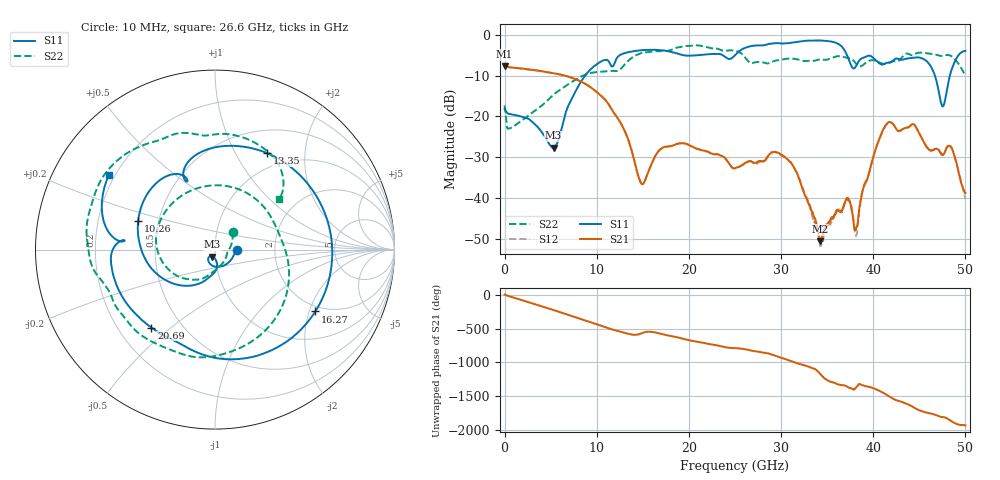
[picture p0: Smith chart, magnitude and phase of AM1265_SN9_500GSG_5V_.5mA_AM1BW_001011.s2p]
!Keysight Technologies,N5245B,MY58422270,A.16.20.02
!Date: Thursday, March 05, 2026 00:38:12
!Correction: S11(C  2-Port  )
!S21(C  2-Port  )
!S12(C  2-Port  )
!S22(C  2-Port  )
!S2P File: Measurements: S11, S21, S12, S22:
# Hz S  dB  R 50
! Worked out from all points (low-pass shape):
!   3201 points, 10 MHz to 50 GHz, reference 50 ohm
!   highest |S21| = -7.68 dB at 10 MHz (marker M1); lowest = -50.6 dB at 34.22 GHz (marker M2)
!   |S21| within 3 dB of the highest: start of sweep to 7.513 GHz
!   lowest |S11| = -27.7 dB at 5.321 GHz (marker M3), VSWR 1.09, Z = 48.4 - j3.74 ohm
!   |S11| at or under -10 dB: start of sweep to 8.743 GHz; 46.69 GHz to 48.31 GHz (1.617 GHz wide, 3.4 % of centre)
!   |S22| runs from -23.0 to -2.6 dB; largest |S21 - S12| = 0.007
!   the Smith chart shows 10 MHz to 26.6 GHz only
!   S11 on the Smith chart (normalised r, x): 10 MHz: 1.28, -0.00; 10.26 GHz: 0.38, +0.15; 13.35 GHz: 0.79, +1.36; 16.27 GHz: 1.82, -2.20; 20.69 GHz: 0.34, -0.43; 26.6 GHz: 0.18, +0.31
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1e7  -18.16 -0.4  -7.68 3.3  -7.65 2.4  -17.28 44.5
2.290794e9  -20.32 -84.1  -8.35 -96.8  -8.36 -96.8  -20.32 -74.6
5.321438e9  -27.67 -111.0  -9.41 134.1  -9.41 134.2  -14.65 -116.9
8.352081e9  -11.27 -132.9  -11.51 -2.7  -11.50 -2.6  -10.16 -172.5
1.025795e10  -6.81 159.8  -14.48 -89.1  -14.47 -89.2  -9.05 125.2
1.335108e10  -4.28 61.5  -25.22 145.3  -25.26 145.3  -6.52 -33.2
1.488202e10  -3.76 10.8  -36.54 150.3  -36.46 150.3  -4.38 -96.3
1.627237e10  -3.65 -31.6  -30.06 165.6  -30.01 166.1  -3.99 -133.6
1.667854e10  -3.69 -43.4  -28.58 153.0  -28.54 153.4  -4.02 -142.3
2.069336e10  -5.03 -129.2  -27.75 30.3  -27.75 30.6  -2.57 148.4
2.5005e10  -4.97 173.6  -32.72 -68.3  -32.65 -69.0  -3.90 71.2
2.659843e10  -2.83 145.1  -30.94 -99.8  -30.98 -99.4  -6.80 38.4
3.066012e10  -2.06 78.5  -30.42 120.2  -30.41 120.6  -5.85 -54.7
3.334708e10  -1.39 35.6  -43.33 -2.0  -44.17 -2.9  -6.35 -127.9
3.422191e10  -1.38 20.5  -50.56 -85.5  -51.05 -79.2  -6.01 -146.3
3.717444e10  -5.08 -41.1  -40.04 82.4  -40.52 82.0  -5.63 156.4
3.815862e10  -7.57 -22.8  -47.26 71.3  -49.12 63.0  -7.14 139.3
4.167354e10  -6.82 -54.6  -21.38 -57.5  -21.35 -57.7  -6.82 114.2
4.511035e10  -5.61 -102.6  -24.60 86.8  -24.65 86.5  -4.35 75.0
4.654757e10  -9.09 -152.5  -28.13 35.0  -28.24 34.5  -4.73 53.8
4.770358e10  -16.86 70.8  -29.09 -10.7  -28.93 -11.4  -5.03 40.7
5e10  -3.91 -73.6  -38.74 -131.5  -40.23 -110.1  -9.79 5.0
